| IBIS file stm32l0_71_72_73_81_82_83_lqfp32.ibs
| Created by s2ibis version 1.1 (customized version)
| North Carolina State University, ERL, 2006
[IBIS ver] 4.2
[File name] stm32l0_71_72_73_81_82_83_lqfp32.ibs
[File Rev] 1.0
[Date]  14-03-2016
[Source] Data Created at STMicroelectronics
[Notes]  File originated from ELDO simulations.
[Disclaimer]  This information is for modeling purpose only and is
   not guaranted. The information is subject to change without
   notice.
[Copyright] Copyright 2016 STMicroelectronics Inc.
|   Component stm32l0_71_72_73_81_82_83_lqfp32
[Component] stm32l0_71_72_73_81_82_83_lqfp32
[Manufacturer] STMicroelectronics
[Package]
| variable   typ   min   max
R_pkg   0.0   0.0   0.0
L_pkg   0.0H   0.0H   0.0H
C_pkg   0.0F   0.0F   0.0F
[Pin]  signal_name   model_name   R_pin   L_pin   C_pin
2 PC14-OSC32_IN io8p_wsudq_ls_ft_v33   54.988E-3   1.7405E-9   14.587E-15
3 PC15-OSC32_OUT io8p_sudq_ls_tc_esdft 53.017E-3   1.6595E-9   8.197E-15
4 NRST ioreset_ft_v33   54.033E-3   1.6554E-9   7.363E-15
5 VDDA POWER   56.223E-3   1.7156E-9   10.783E-15
6 PA0 io8p_wsudq_ls_ft_v33   61.160E-3   1.8629E-9   10.243E-15
7 PA1 io8p_wsudq_lcd4_ls_ft  59.987E-3   1.8648E-9   10.852E-15
8 PA2 io8p_wsudq_lcd4_ls_ft  71.192E-3   2.1932E-9   17.019E-15
9 PA3 io8p_wsudq_lcd4_ls_ft  71.059E-3   2.1776E-9   16.855E-15
10 PA4 io8p_wsudq_i2cin_ls_ft 63.005E-3   1.9478E-9   14.439E-15
11 PA5 io8p_wsudq_i2cin_ls_ft  58.243E-3   1.7981E-9   7.948E-15
12 PA6 io8p_wsudq_lcd4_ls_ft  55.874E-3   1.7092E-9   8.812E-15
13 PA7 io8p_wsudq_lcd4_ls_ft  55.141E-3   1.6964E-9   12.212E-15
14 PB0 io8p_wsudq_lcd4_ls_ft  56.661E-3   1.7554E-9   4.706E-15
15 PB1 io8p_wsudq_lcd4_ls_ft  61.182E-3   1.8979E-9   13.557E-15
16 VSS GND   68.639E-3   2.1172E-9   16.500E-15
17 VDD POWER   66.539E-3   2.0692E-9   17.677E-15
18 PA8 io8p_sudq_lcd4_i2cin_ls_ft   71.158E-3   2.1438E-9   11.062E-15
19 PA9 io8p_sudq_lcd4_i2cin_ls_ft   63.842E-3   1.9327E-9   9.196E-15
20 PA10 io8p_sudq_lcd4_i2cin_ls_ft   58.291E-3   1.7635E-9   11.677E-15
21 PA11 io8usb_ls_ft   54.700E-3   1.6700E-9   6.891E-15
22 PA12 io8usb_ls_ft   53.046E-3   1.6525E-9   10.905E-15
23 PA13 io8p_sudq_ls_ft   62.866E-3   1.9450E-9   11.111E-15
24 PA14 io8p_sudq_ls_ft   75.711E-3   2.3060E-9   17.278E-15
25 PA15 io8p_wsudq_lcd4_ls_ft   74.224E-3   2.2583E-9   19.736E-15
26 PB3 io8p_wsudq_lcd4_ls_ft   65.224E-3   2.0006E-9   8.439E-15
27 PB4 io8p_sudq_lcd4_i2cin_ls_ft 59.281E-3   1.8183E-9   10.281E-15
28 PB5 io8p_wsudq_lcd4_ls_ft   56.029E-3   1.7169E-9   8.461E-15
29 PB6 io8p_wsudq_i2cin_ls_ft   55.139E-3   1.6969E-9   12.383E-15
30 PB7 io8p_wsudq_i2cin_ls_ft   56.372E-3   1.7463E-9   4.202E-15
31 BOOT0 vpp_test_hv  59.845E-3   1.8672E-9   13.676E-15
32 VSS GND   66.777E-3   2.0705E-9   14.725E-15
1 VDD POWER   64.896E-3   2.0240E-9   16.235E-15
[Model Selector] io8p_sudq_ls_ft
io8p00_sudq_ls_ft_pd_lv  "SPEED00 1P8V, PD=40kOhm"
io8p00_sudq_ls_ft_pu_lv  "SPEED00 1P8V, PU=40kOhm"
io8p00_sudq_ls_ft_lv  "SPEED00 1P8V"
io8p01_sudq_ls_ft_pd_lv  "SPEED01 1P8V, PD=40kOhm"
io8p01_sudq_ls_ft_pu_lv  "SPEED01 1P8V, PU=40kOhm"
io8p01_sudq_ls_ft_lv  "SPEED01 1P8V"
io8p10_sudq_ls_ft_pd_lv  "SPEED10 1P8V, PD=40kOhm"
io8p10_sudq_ls_ft_pu_lv  "SPEED10 1P8V, PU=40kOhm"
io8p10_sudq_ls_ft_lv  "SPEED10 1P8V"
io8p11_sudq_ls_ft_pd_lv  "SPEED11 1P8V, PD=40kOhm"
io8p11_sudq_ls_ft_pu_lv  "SPEED11 1P8V, PU=40kOhm"
io8p11_sudq_ls_ft_lv  "SPEED11 1P8V"
io8p00_sudq_ls_ft_pd  "SPEED00, PD=40kOhm"
io8p00_sudq_ls_ft_pu  "SPEED00, PU=40kOhm"
io8p00_sudq_ls_ft  "SPEED00"
io8p01_sudq_ls_ft_pd  "SPEED01, PD=40kOhm"
io8p01_sudq_ls_ft_pu  "SPEED01, PU=40kOhm"
io8p01_sudq_ls_ft  "SPEED01"
io8p10_sudq_ls_ft_pd  "SPEED10, PD=40kOhm"
io8p10_sudq_ls_ft_pu  "SPEED10, PU=40kOhm"
io8p10_sudq_ls_ft  "SPEED10"
io8p11_sudq_ls_ft_pd  "SPEED11, PD=40kOhm"
io8p11_sudq_ls_ft_pu  "SPEED11, PU=40kOhm"
io8p11_sudq_ls_ft  "SPEED11"
[Model Selector] io8p_sudq_ls_tc_esdft
io8p00_sudq_ls_tc_esdft_pd_lv  "SPEED00 1P8V, PD=40kOhm"
io8p00_sudq_ls_tc_esdft_pu_lv  "SPEED00 1P8V, PU=40kOhm"
io8p00_sudq_ls_tc_esdft_lv  "SPEED00 1P8V"
io8p01_sudq_ls_tc_esdft_pd_lv  "SPEED01 1P8V, PD=40kOhm"
io8p01_sudq_ls_tc_esdft_pu_lv  "SPEED01 1P8V, PU=40kOhm"
io8p01_sudq_ls_tc_esdft_lv  "SPEED01 1P8V"
io8p10_sudq_ls_tc_esdft_pd_lv  "SPEED10 1P8V, PD=40kOhm"
io8p10_sudq_ls_tc_esdft_pu_lv  "SPEED10 1P8V, PU=40kOhm"
io8p10_sudq_ls_tc_esdft_lv  "SPEED10 1P8V"
io8p11_sudq_ls_tc_esdft_pd_lv  "SPEED11 1P8V, PD=40kOhm"
io8p11_sudq_ls_tc_esdft_pu_lv  "SPEED11 1P8V, PU=40kOhm"
io8p11_sudq_ls_tc_esdft_lv  "SPEED11 1P8V"
io8p00_sudq_ls_tc_esdft_pd  "SPEED00, PD=40kOhm"
io8p00_sudq_ls_tc_esdft_pu  "SPEED00, PU=40kOhm"
io8p00_sudq_ls_tc_esdft  "SPEED00"
io8p01_sudq_ls_tc_esdft_pd  "SPEED01, PD=40kOhm"
io8p01_sudq_ls_tc_esdft_pu  "SPEED01, PU=40kOhm"
io8p01_sudq_ls_tc_esdft  "SPEED01"
io8p10_sudq_ls_tc_esdft_pd  "SPEED10, PD=40kOhm"
io8p10_sudq_ls_tc_esdft_pu  "SPEED10, PU=40kOhm"
io8p10_sudq_ls_tc_esdft  "SPEED10"
io8p11_sudq_ls_tc_esdft_pd  "SPEED11, PD=40kOhm"
io8p11_sudq_ls_tc_esdft_pu  "SPEED11, PU=40kOhm"
io8p11_sudq_ls_tc_esdft  "SPEED11"
[Model Selector] io8p_wsudq_i2cin_ls_ft
io8p00_wsudq_i2cin_ls_ft_pd_lv  "SPEED00 1P8V, PD=40kOhm"
io8p00_wsudq_i2cin_ls_ft_pu_lv  "SPEED00 1P8V, PU=40kOhm"
io8p00_wsudq_i2cin_ls_ft_lv  "SPEED00 1P8V"
io8p01_wsudq_i2cin_ls_ft_pd_lv  "SPEED01 1P8V, PD=40kOhm"
io8p01_wsudq_i2cin_ls_ft_pu_lv  "SPEED01 1P8V, PU=40kOhm"
io8p01_wsudq_i2cin_ls_ft_lv  "SPEED01 1P8V"
io8p10_wsudq_i2cin_ls_ft_pd_lv  "SPEED10 1P8V, PD=40kOhm"
io8p10_wsudq_i2cin_ls_ft_pu_lv  "SPEED10 1P8V, PU=40kOhm"
io8p10_wsudq_i2cin_ls_ft_lv  "SPEED10 1P8V"
io8p11_wsudq_i2cin_ls_ft_pd_lv  "SPEED11 1P8V, PD=40kOhm"
io8p11_wsudq_i2cin_ls_ft_pu_lv  "SPEED11 1P8V, PU=40kOhm"
io8p11_wsudq_i2cin_ls_ft_lv  "SPEED11 1P8V"
io8p00_wsudq_i2cin_ls_ft_pd  "SPEED00, PD=40kOhm"
io8p00_wsudq_i2cin_ls_ft_pu  "SPEED00, PU=40kOhm"
io8p00_wsudq_i2cin_ls_ft  "SPEED00"
io8p01_wsudq_i2cin_ls_ft_pd  "SPEED01, PD=40kOhm"
io8p01_wsudq_i2cin_ls_ft_pu  "SPEED01, PU=40kOhm"
io8p01_wsudq_i2cin_ls_ft  "SPEED01"
io8p10_wsudq_i2cin_ls_ft_pd  "SPEED10, PD=40kOhm"
io8p10_wsudq_i2cin_ls_ft_pu  "SPEED10, PU=40kOhm"
io8p10_wsudq_i2cin_ls_ft  "SPEED10"
io8p11_wsudq_i2cin_ls_ft_pd  "SPEED11, PD=40kOhm"
io8p11_wsudq_i2cin_ls_ft_pu  "SPEED11, PU=40kOhm"
io8p11_wsudq_i2cin_ls_ft  "SPEED11"
[Model Selector] io8p_wsudq_lcd4_ls_ft
io8p00_wsudq_lcd4_ls_ft_pd_lv  "SPEED00 1P8V, PD=40kOhm"
io8p00_wsudq_lcd4_ls_ft_pu_lv  "SPEED00 1P8V, PU=40kOhm"
io8p00_wsudq_lcd4_ls_ft_lv  "SPEED00 1P8V"
io8p01_wsudq_lcd4_ls_ft_pd_lv  "SPEED01 1P8V, PD=40kOhm"
io8p01_wsudq_lcd4_ls_ft_pu_lv  "SPEED01 1P8V, PU=40kOhm"
io8p01_wsudq_lcd4_ls_ft_lv  "SPEED01 1P8V"
io8p10_wsudq_lcd4_ls_ft_pd_lv  "SPEED10 1P8V, PD=40kOhm"
io8p10_wsudq_lcd4_ls_ft_pu_lv  "SPEED10 1P8V, PU=40kOhm"
io8p10_wsudq_lcd4_ls_ft_lv  "SPEED10 1P8V"
io8p11_wsudq_lcd4_ls_ft_pd_lv  "SPEED11 1P8V, PD=40kOhm"
io8p11_wsudq_lcd4_ls_ft_pu_lv  "SPEED11 1P8V, PU=40kOhm"
io8p11_wsudq_lcd4_ls_ft_lv  "SPEED11 1P8V"
io8p00_wsudq_lcd4_ls_ft_pd  "SPEED00, PD=40kOhm"
io8p00_wsudq_lcd4_ls_ft_pu  "SPEED00, PU=40kOhm"
io8p00_wsudq_lcd4_ls_ft  "SPEED00"
io8p01_wsudq_lcd4_ls_ft_pd  "SPEED01, PD=40kOhm"
io8p01_wsudq_lcd4_ls_ft_pu  "SPEED01, PU=40kOhm"
io8p01_wsudq_lcd4_ls_ft  "SPEED01"
io8p10_wsudq_lcd4_ls_ft_pd  "SPEED10, PD=40kOhm"
io8p10_wsudq_lcd4_ls_ft_pu  "SPEED10, PU=40kOhm"
io8p10_wsudq_lcd4_ls_ft  "SPEED10"
io8p11_wsudq_lcd4_ls_ft_pd  "SPEED11, PD=40kOhm"
io8p11_wsudq_lcd4_ls_ft_pu  "SPEED11, PU=40kOhm"
io8p11_wsudq_lcd4_ls_ft  "SPEED11"
[Model Selector] io8p_wsudq_ls_ft_v33
io8p00_wsudq_ls_ft_v33_pd_lv  "SPEED00 1P8V, PD=40kOhm"
io8p00_wsudq_ls_ft_v33_pu_lv  "SPEED00 1P8V, PU=40kOhm"
io8p00_wsudq_ls_ft_v33_lv  "SPEED00 1P8V"
io8p01_wsudq_ls_ft_v33_pd_lv  "SPEED01 1P8V, PD=40kOhm"
io8p01_wsudq_ls_ft_v33_pu_lv  "SPEED01 1P8V, PU=40kOhm"
io8p01_wsudq_ls_ft_v33_lv  "SPEED01 1P8V"
io8p10_wsudq_ls_ft_v33_pd_lv  "SPEED10 1P8V, PD=40kOhm"
io8p10_wsudq_ls_ft_v33_pu_lv  "SPEED10 1P8V, PU=40kOhm"
io8p10_wsudq_ls_ft_v33_lv  "SPEED10 1P8V"
io8p11_wsudq_ls_ft_v33_pd_lv  "SPEED11 1P8V, PD=40kOhm"
io8p11_wsudq_ls_ft_v33_pu_lv  "SPEED11 1P8V, PU=40kOhm"
io8p11_wsudq_ls_ft_v33_lv  "SPEED11 1P8V"
io8p00_wsudq_ls_ft_v33_pd  "SPEED00, PD=40kOhm"
io8p00_wsudq_ls_ft_v33_pu  "SPEED00, PU=40kOhm"
io8p00_wsudq_ls_ft_v33  "SPEED00"
io8p01_wsudq_ls_ft_v33_pd  "SPEED01, PD=40kOhm"
io8p01_wsudq_ls_ft_v33_pu  "SPEED01, PU=40kOhm"
io8p01_wsudq_ls_ft_v33  "SPEED01"
io8p10_wsudq_ls_ft_v33_pd  "SPEED10, PD=40kOhm"
io8p10_wsudq_ls_ft_v33_pu  "SPEED10, PU=40kOhm"
io8p10_wsudq_ls_ft_v33  "SPEED10"
io8p11_wsudq_ls_ft_v33_pd  "SPEED11, PD=40kOhm"
io8p11_wsudq_ls_ft_v33_pu  "SPEED11, PU=40kOhm"
io8p11_wsudq_ls_ft_v33  "SPEED11"
[Model Selector] vpp_test_hv
vpp_test_hv_2p4  "Input Buffer 1P65V"
vpp_test_hv_3p3  "Input Buffer"
[Model Selector] io8usb_ls_ft
io8usb_ls_ft_dpdn_pu  "HS USB DP/DN IO + PU=1.2kOhm"
io8usb_ls_ft_dpdn  "HS USB DP/DN IO"
io8p00_ls_ft_pd_lv  "SPEED00 1P8V, PD=40kOhm"
io8p00_ls_ft_pu_lv  "SPEED00 1P8V, PU=40kOhm"
io8p00_ls_ft_lv  "SPEED00 1P8V"
io8p01_ls_ft_pd_lv  "SPEED01 1P8V, PD=40kOhm"
io8p01_ls_ft_pu_lv  "SPEED01 1P8V, PU=40kOhm"
io8p01_ls_ft_lv  "SPEED01 1P8V"
io8p10_ls_ft_pd_lv  "SPEED10 1P8V, PD=40kOhm"
io8p10_ls_ft_pu_lv  "SPEED10 1P8V, PU=40kOhm"
io8p10_ls_ft_lv  "SPEED10 1P8V"
io8p11_ls_ft_pd_lv  "SPEED11 1P8V, PD=40kOhm"
io8p11_ls_ft_pu_lv  "SPEED11 1P8V, PU=40kOhm"
io8p11_ls_ft_lv  "SPEED11 1P8V"
io8p00_ls_ft_pd  "SPEED00, PD=40kOhm"
io8p00_ls_ft_pu  "SPEED00, PU=40kOhm"
io8p00_ls_ft  "SPEED00"
io8p01_ls_ft_pd  "SPEED01, PD=40kOhm"
io8p01_ls_ft_pu  "SPEED01, PU=40kOhm"
io8p01_ls_ft  "SPEED01"
io8p10_ls_ft_pd  "SPEED10, PD=40kOhm"
io8p10_ls_ft_pu  "SPEED10, PU=40kOhm"
io8p10_ls_ft  "SPEED10"
io8p11_ls_ft_pd  "SPEED11, PD=40kOhm"
io8p11_ls_ft_pu  "SPEED11, PU=40kOhm"
io8p11_ls_ft  "SPEED11"
[Model Selector] io8p_sudq_lcd4_i2cin_ls_ft
io8p00_sudq_lcd4_i2cin_ls_ft_pd_lv  "SPEED00 1P8V, PD=40kOhm"
io8p00_sudq_lcd4_i2cin_ls_ft_pu_lv  "SPEED00 1P8V, PU=40kOhm"
io8p00_sudq_lcd4_i2cin_ls_ft_lv  "SPEED00 1P8V"
io8p01_sudq_lcd4_i2cin_ls_ft_pd_lv  "SPEED01 1P8V, PD=40kOhm"
io8p01_sudq_lcd4_i2cin_ls_ft_pu_lv  "SPEED01 1P8V, PU=40kOhm"
io8p01_sudq_lcd4_i2cin_ls_ft_lv  "SPEED01 1P8V"
io8p10_sudq_lcd4_i2cin_ls_ft_pd_lv  "SPEED10 1P8V, PD=40kOhm"
io8p10_sudq_lcd4_i2cin_ls_ft_pu_lv  "SPEED10 1P8V, PU=40kOhm"
io8p10_sudq_lcd4_i2cin_ls_ft_lv  "SPEED10 1P8V"
io8p11_sudq_lcd4_i2cin_ls_ft_pd_lv  "SPEED11 1P8V, PD=40kOhm"
io8p11_sudq_lcd4_i2cin_ls_ft_pu_lv  "SPEED11 1P8V, PU=40kOhm"
io8p11_sudq_lcd4_i2cin_ls_ft_lv  "SPEED11 1P8V"
io8p00_sudq_lcd4_i2cin_ls_ft_pd  "SPEED00, PD=40kOhm"
io8p00_sudq_lcd4_i2cin_ls_ft_pu  "SPEED00, PU=40kOhm"
io8p00_sudq_lcd4_i2cin_ls_ft  "SPEED00"
io8p01_sudq_lcd4_i2cin_ls_ft_pd  "SPEED01, PD=40kOhm"
io8p01_sudq_lcd4_i2cin_ls_ft_pu  "SPEED01, PU=40kOhm"
io8p01_sudq_lcd4_i2cin_ls_ft  "SPEED01"
io8p10_sudq_lcd4_i2cin_ls_ft_pd  "SPEED10, PD=40kOhm"
io8p10_sudq_lcd4_i2cin_ls_ft_pu  "SPEED10, PU=40kOhm"
io8p10_sudq_lcd4_i2cin_ls_ft  "SPEED10"
io8p11_sudq_lcd4_i2cin_ls_ft_pd  "SPEED11, PD=40kOhm"
io8p11_sudq_lcd4_i2cin_ls_ft_pu  "SPEED11, PU=40kOhm"
io8p11_sudq_lcd4_i2cin_ls_ft  "SPEED11"
[Model Selector] ioreset_ft_v33
ioreset_ft_v33_pu_lv  "ioreset 1P8V + PU=40kOhm"
ioreset_ft_v33_nopu_lv  "ioreset 1P8V"
ioreset_ft_v33_pu  "ioreset + PU=40kOhm"
ioreset_ft_v33_nopu  "ioreset"
| Models and submodels in the file (176): io8p00_sudq_ls_ft_pd_lv (I/O), io8p00_sudq_ls_ft_pu_lv (I/O), io8p00_sudq_ls_ft_lv (I/O), io8p01_sudq_ls_ft_pd_lv (I/O), io8p01_sudq_ls_ft_pu_lv (I/O), io8p01_sudq_ls_ft_lv (I/O), io8p10_sudq_ls_ft_pd_lv (I/O), io8p10_sudq_ls_ft_pu_lv (I/O), io8p10_sudq_ls_ft_lv (I/O), io8p11_sudq_ls_ft_pd_lv (I/O), io8p11_sudq_ls_ft_pu_lv (I/O), io8p11_sudq_ls_ft_lv (I/O), io8p00_sudq_ls_ft_pd (I/O), io8p00_sudq_ls_ft_pu (I/O), io8p00_sudq_ls_ft (I/O), io8p01_sudq_ls_ft_pd (I/O), io8p01_sudq_ls_ft_pu (I/O), io8p01_sudq_ls_ft (I/O), io8p10_sudq_ls_ft_pd (I/O), io8p10_sudq_ls_ft_pu (I/O), io8p10_sudq_ls_ft (I/O), io8p11_sudq_ls_ft_pd (I/O), io8p11_sudq_ls_ft_pu (I/O), io8p11_sudq_ls_ft (I/O), io8p00_sudq_ls_tc_esdft_pd_lv (I/O), io8p00_sudq_ls_tc_esdft_pu_lv (I/O), io8p00_sudq_ls_tc_esdft_lv (I/O), io8p01_sudq_ls_tc_esdft_pd_lv (I/O), io8p01_sudq_ls_tc_esdft_pu_lv (I/O), io8p01_sudq_ls_tc_esdft_lv (I/O), io8p10_sudq_ls_tc_esdft_pd_lv (I/O), io8p10_sudq_ls_tc_esdft_pu_lv (I/O), io8p10_sudq_ls_tc_esdft_lv (I/O), io8p11_sudq_ls_tc_esdft_pd_lv (I/O), io8p11_sudq_ls_tc_esdft_pu_lv (I/O), io8p11_sudq_ls_tc_esdft_lv (I/O), io8p00_sudq_ls_tc_esdft_pd (I/O), io8p00_sudq_ls_tc_esdft_pu (I/O), io8p00_sudq_ls_tc_esdft (I/O), io8p01_sudq_ls_tc_esdft_pd (I/O), io8p01_sudq_ls_tc_esdft_pu (I/O), io8p01_sudq_ls_tc_esdft (I/O), io8p10_sudq_ls_tc_esdft_pd (I/O), io8p10_sudq_ls_tc_esdft_pu (I/O), io8p10_sudq_ls_tc_esdft (I/O), io8p11_sudq_ls_tc_esdft_pd (I/O), io8p11_sudq_ls_tc_esdft_pu (I/O), io8p11_sudq_ls_tc_esdft (I/O), io8p00_wsudq_i2cin_ls_ft_pd_lv (I/O), io8p00_wsudq_i2cin_ls_ft_pu_lv (I/O), io8p00_wsudq_i2cin_ls_ft_lv (I/O), io8p01_wsudq_i2cin_ls_ft_pd_lv (I/O), io8p01_wsudq_i2cin_ls_ft_pu_lv (I/O), io8p01_wsudq_i2cin_ls_ft_lv (I/O), io8p10_wsudq_i2cin_ls_ft_pd_lv (I/O), io8p10_wsudq_i2cin_ls_ft_pu_lv (I/O), io8p10_wsudq_i2cin_ls_ft_lv (I/O), io8p11_wsudq_i2cin_ls_ft_pd_lv (I/O), io8p11_wsudq_i2cin_ls_ft_pu_lv (I/O), io8p11_wsudq_i2cin_ls_ft_lv (I/O), io8p00_wsudq_i2cin_ls_ft_pd (I/O), io8p00_wsudq_i2cin_ls_ft_pu (I/O), io8p00_wsudq_i2cin_ls_ft (I/O), io8p01_wsudq_i2cin_ls_ft_pd (I/O), io8p01_wsudq_i2cin_ls_ft_pu (I/O), io8p01_wsudq_i2cin_ls_ft (I/O), io8p10_wsudq_i2cin_ls_ft_pd (I/O), io8p10_wsudq_i2cin_ls_ft_pu (I/O), io8p10_wsudq_i2cin_ls_ft (I/O), io8p11_wsudq_i2cin_ls_ft_pd (I/O), io8p11_wsudq_i2cin_ls_ft_pu (I/O), io8p11_wsudq_i2cin_ls_ft (I/O), io8p00_wsudq_lcd4_ls_ft_pd_lv (I/O), io8p00_wsudq_lcd4_ls_ft_pu_lv (I/O), io8p00_wsudq_lcd4_ls_ft_lv (I/O), io8p01_wsudq_lcd4_ls_ft_pd_lv (I/O), io8p01_wsudq_lcd4_ls_ft_pu_lv (I/O), io8p01_wsudq_lcd4_ls_ft_lv (I/O), io8p10_wsudq_lcd4_ls_ft_pd_lv (I/O), io8p10_wsudq_lcd4_ls_ft_pu_lv (I/O)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
